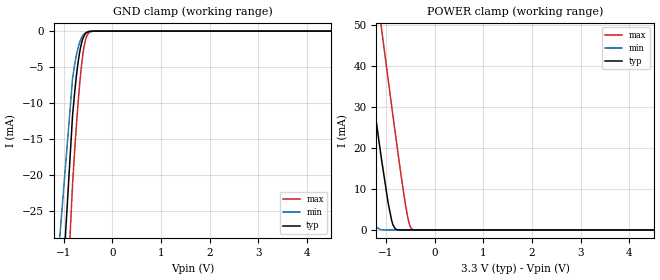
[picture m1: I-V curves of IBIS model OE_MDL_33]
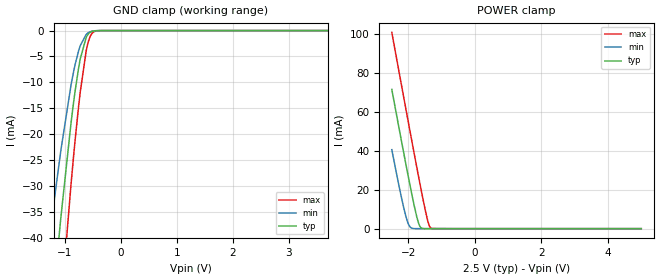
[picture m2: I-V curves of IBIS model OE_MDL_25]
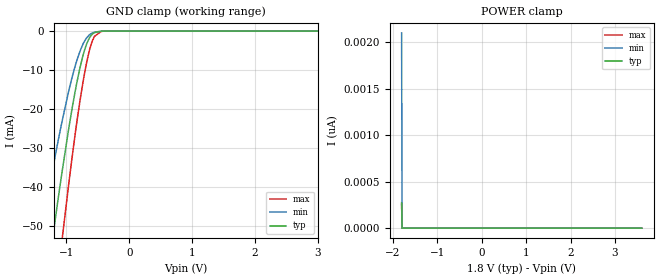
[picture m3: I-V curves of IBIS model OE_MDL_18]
|Texas Instruments Incorporated
| Put part description here: I2C Translator w/ independent A & B side supplies
| Marketing Part # : TCA9416DTM
| Digital Voltage Range : 1.08V-3.6V
| Package-type: DTM
| #pins/pkg drawing : 8-pin
[IBIS Ver]   4.1
[File name]   tca9416.ibs
[Date]   08/2020
[File Rev]   1.0
[Source]
| Texas Instruments Incorporated.
| 12500 TI Blvd
| Dallas, TX 75243
[Notes]
[Disclaimer]  provided as is
[Copyright]   Copyright 2020 IO Methodology Inc. All rights reserved.
|   COMPONENT: TCA9416DTM
[Component]   TCA9416DTM
[Manufacturer]  Texas Instruments Incorporated
[Package]
|   typ   min   max
R_pkg   0.04   0.03   0.05
L_pkg   0.4nH   0.3nH   0.5nH
C_pkg   0.3pF   0.07pF   0.8pF
[Pin]  signal_name  model_name   R_pin   L_pin   C_pin
1   SCL_A   I2C_MDL   0.032   0.28nH   0.07pF
2   OE   OE_MDL   0.031   0.27nH   0.31pF
3   VCCA   POWER   0.032   0.29nH   0.07pF
4   SDA_A   I2C_MDL   0.040   0.41nH   0.79pF
5   SDA_B   I2C_MDL   0.032   0.28nH   0.07pF
6   VSSA   GND   0.031   0.27nH   0.07pF
7   VCCB   I2C_MDL   0.032   0.29nH   0.31pF
8   SCL_B   I2C_MDL   0.040   0.41nH   0.79pF
| Model I2C_MDL
[Model Selector]   I2C_MDL
I2C_MDL_33   3.3 volt Vcc
I2C_MDL_25   2.5 volt Vcc
I2C_MDL_18   1.8 volt Vcc
I2C_MDL_12   1.2 volt Vcc
| Model OE_MDL
[Model Selector]   OE_MDL
OE_MDL_33   3.3 volt Vcc
OE_MDL_25   2.5 volt Vcc
OE_MDL_18   1.8 volt Vcc
OE_MDL_12   1.2 volt Vcc
| Models and submodels in the file (8): OE_MDL_33 (Input), OE_MDL_25 (Input), OE_MDL_18 (Input), OE_MDL_12 (Input), I2C_MDL_33 (I/O), I2C_MDL_25 (I/O), I2C_MDL_18 (I/O), I2C_MDL_12 (I/O)
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[Model]   OE_MDL_33
Model_type   Input
Vinl = 1.155
Vinh = 2.145
|   typ   min   max
C_comp   2pF   1.95pF   2.13pF
[Voltage Range]   3.3   3   3.6
[Temperature Range]   27   125   -40
[Power Clamp Reference]   3.3   3   3.6
[GND Clamp Reference]   0   0   0
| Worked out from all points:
|   GND clamp passes 1 mA (typ) near -0.60 V on its own axis
|   POWER clamp passes 1 mA (typ) near -0.85 V on its own axis
[GND Clamp]
|   Voltage   I(typ)   I(min)   I(max)
-3.3V     -1.372A    -589.8mA   -1.96A
-1.617V   -103mA     -73.77mA   -133.6mA
-815.1mV  -11.73mA   -6.589mA   -21.23mA
-735.9mV  -6.225mA   -3.328mA   -13.08mA
-656.7mV  -2.469mA   -1.325mA   -6.464mA
-617.1mV  -1.336mA   -756.1uA   -3.957mA
-587.4mV  -781.3uA   -474.7uA   -2.514mA
-557.7mV  -429.1uA   -286.8uA   -1.465mA
-518.1mV  -177.2uA   -138uA     -619.7uA
-458.7mV  -40.4uA    -40.48uA   -131.5uA
-320.1mV  -667nA     -1.501uA   -1.119uA
6.6V      0A         0A         0A
[POWER Clamp]
|   Voltage   I(typ)   I(min)   I(max)
-3.3V     221.1mA    183.3mA    256.2mA
-1.973V   96.81mA    60.54mA    131.1mA
-1.627V   64.8mA     29.85mA    98.65mA
-1.498V   53.03mA    19.06mA    86.65mA
-1.399V   44.06mA    11.33mA    77.43mA
-1.28V    33.43mA    3.683mA    66.41mA
-1.132V   20.49mA    143.5uA    52.71mA
-1.092V   17.15mA    46.6uA     49.08mA
-854.7mV  1.161mA    35nA       27.55mA
-577.5mV  27nA       0A         4.584mA
-458.7mV  0A         0A         127.2uA
6.6V      0A         0A         0A
[Model]   OE_MDL_25
Model_type   Input
Vinl = 0.875
Vinh = 1.625
|   typ   min   max
C_comp   2pF   1.95pF   2.13pF
[Voltage Range]   2.5   2.25   2.75
[Temperature Range]   27   125   -40
[Power Clamp Reference]   2.5   2.25   2.75
[GND Clamp Reference]   0   0   0
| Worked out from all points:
|   GND clamp passes 1 mA (typ) near -0.60 V on its own axis
|   POWER clamp passes 1 mA (typ) near -1.65 V on its own axis
[GND Clamp]
|OE_MDL_25
|   Voltage   I(typ)   I(min)   I(max)
-2.5V     -219.3mA   -169.8mA   -448.1mA
-1.255V   -57.53mA   -38.78mA   -79.99mA
-1.165V   -46.92mA   -30.95mA   -67.03mA
-1.075V   -36.78mA   -23.62mA   -54.38mA
-1.067V   -35.96mA   -23.04mA   -53.34mA
-887.5mV  -17.85mA   -10.52mA   -29.7mA
-752.5mV  -7.251mA   -3.91mA    -14.68mA
-617.5mV  -1.345mA   -760.7uA   -3.979mA
-557.5mV  -427.3uA   -285.8uA   -1.459mA
-482.5mV  -74.59uA   -67.38uA   -253uA
-362.5mV  -2.57uA    -4.314uA   -5.763uA
5V        0A         0A         0A
[POWER Clamp]
|OE_MDL_25
|   Voltage   I(typ)   I(min)   I(max)
-2.5V     71.51mA    40.57mA    100.8mA
-2.147V   39.41mA    11.2mA     67.99mA
-2.08V    33.39mA    6.534mA    61.75mA
-1.99V    25.48mA    1.936mA    53.46mA
-1.907V   18.43mA    289.4uA    45.89mA
-1.758V   6.651mA    3.98uA     32.28mA
-1.667V   1.595mA    281.5nA    24.25mA
-1.593V   157.4uA    24.23nA    17.71mA
-1.435V   369.2nA    0A         5.095mA
-1.375V   26.27nA    0A         1.599mA
-1.323V   0A         0A         238.6uA
5V        0A         0A         0A
[Model]   OE_MDL_18
Model_type   Input
Vinl = 0.630
Vinh = 1.170
|   typ   min   max
C_comp   2pF   1.95pF   2.13pF
[Voltage Range]   1.8   1.62   1.98
[Temperature Range]   27   125   -40
[Power Clamp Reference]   1.8   1.62   1.98
[GND Clamp Reference]   0   0   0
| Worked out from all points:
|   GND clamp passes 1 mA (typ) near -0.60 V on its own axis
[GND Clamp]
|OE_MDL_18
|   Voltage   I(typ)   I(min)   I(max)
-1.8V     -126.9mA   -92.88mA   -161mA
-1.325V   -66mA      -45.13mA   -90.19mA
-1.26V    -58.13mA   -39.23mA   -80.71mA
-1.184V   -49.17mA   -32.6mA    -69.8mA
-1.076V   -36.93mA   -23.73mA   -54.57mA
-914.4mV  -20.33mA   -12.17mA   -33.04mA
-784.8mV  -9.449mA   -5.199mA   -17.96mA
-682.2mV  -3.462mA   -1.835mA   -8.387mA
-606.6mV  -1.114mA   -644.2uA   -3.402mA
-552.6mV  -384.9uA   -262uA     -1.323mA
-401.4mV  -8.249uA   -10.97uA   -22.58uA
3.6V      0A         0A         0A
[POWER Clamp]
|OE_MDL_18
|   Voltage   I(typ)   I(min)   I(max)
-1.8V     275.2pA    2.103nA    256.6pA
-1.789V   0A         0A         0A
-1.784V   0A         0A         0A
3.6V      0A         0A         0A
